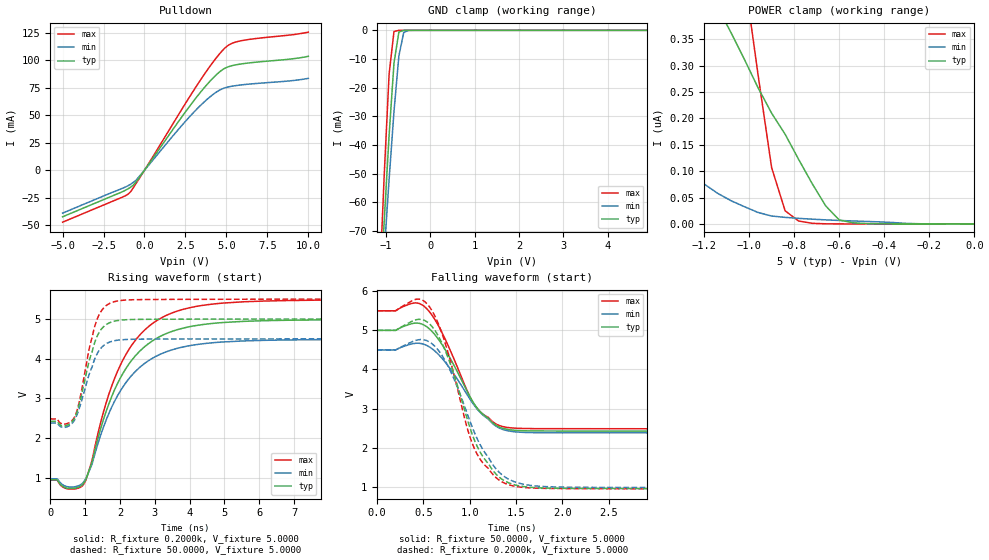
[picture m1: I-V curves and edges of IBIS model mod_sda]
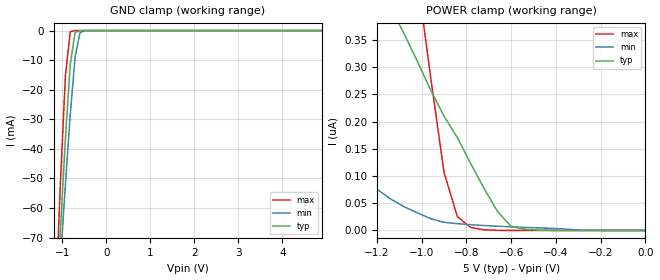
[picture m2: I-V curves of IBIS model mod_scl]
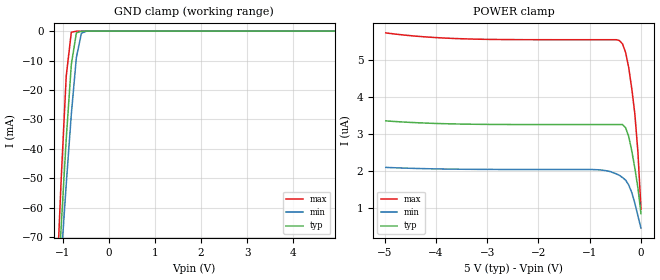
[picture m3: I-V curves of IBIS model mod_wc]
| IBIS (I/O, Buffer, Information, Specification) Model, officially
| electronic behavioral standard for Buffer structures of digital pins.
[IBIS ver]  4.0
[File name] m24512e_5d0_dfn8.ibs
[File Rev]  1.0
[Date]   26 Jan 2023
[Source]   CAD & Design Services (Catania) - STMicroelectronics
[Notes]
   (Note1)  This IBIS model includes the DFN8 package parasitic data
   (Note2)  This IBIS model has some Notes about the non-monotonicity
   of the I-V curves, but they are not indicative of problems
   inside the model;
[Disclaimer]
   Customers are solely responsible for all aspects of their
   own product designs or applications using this IBIS Model.
   STMicroelectronics assumes no liability for Custmer Designs
   and applications associated to this IBIS Model.
   In the use of this IBIS Model Customer shall not modify,
   disassemble, alter this Model in whole or in part.
   If Customers do not accept these terms, the IBIS Model
   may not be used. For any problems or modifications please
   contact STMicroelectronics (www.st.com).
[Copyright] (c) 2023 STMicroelectronics
|   Component M24512E
[Component] M24512E
[Manufacturer] STMicroelectronics
[Package]
| variable  typ   min   max
R_pkg   0.0   0.0   0.0
L_pkg   0.0H   0.0H   0.0H
C_pkg   0.0F   0.0F   0.0F
[Pin]   signal_name   model_name   R_pin   L_pin   C_pin
1   NC   NC   0.0   0.0   0.0
2   NC   NC   0.0   0.0   0.0
3   NC   NC   0.0   0.0   0.0
4   VSS   GND   0.0   0.0   0.0
5   SDA   mod_sda   0.0   0.0   0.0
6   SCL   mod_scl   0.0   0.0   0.0
7   WC   mod_wc   0.0   0.0   0.0
8   VCC   POWER   0.0   0.0   0.0
[Package Model]  182694_DFN8   | also called 182694_MLP_2x3
[Define Package Model]  182694_DFN8
[Manufacturer]  STMicroelectronics
[OEM]  STMicroelectronics
[Description]  8 pin DFN8 2x3
[Number Of Pins]  8
[Pin Numbers]
|Pin Num   Terminal Name
1   | net1
2   | net2
3   | net3
4   | net4_GND
5   | net5
6   | net6
7   | net7
8   | net8_VDD
[Model Data]
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[End Model Data]
[End Package Model]
| Models and submodels in the file (3): mod_sda (I/O_open_drain), mod_scl (Input), mod_wc (Input)
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|   Model mod_sda
[Model]   mod_sda
Model_type I/O_open_drain
Polarity   Inverting
Vinl   =   1.500V
Vinh   =   3.500V
Vmeas  =   2.500V
Cref   =   30pF
Rref   =   500
Vref   =   5.000V
C_comp   4.636pF   4.427pF   4.856pF
[Temperature Range]  25.0000   85.0000   -40.0000
[Voltage Range]   5.0000V   4.5000V   5.5000V
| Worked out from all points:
|   slope of the pulldown table from 0 to 0.75 V, typ, clamps not added: 46.8 ohm
|   GND clamp passes 1 mA (typ) near -0.71 V on its own axis
|   rising waveform, R_fixture 0.2000k, V_fixture 5.0000: 20-80 % time 1.26ns typ, 1.27ns min, 1.26ns max; typ from 0.947 V to 4.99 V
|   rising waveform, R_fixture 50.0000, V_fixture 5.0000: 20-80 % time 451ps typ, 465ps min, 432ps max; typ from 2.42 V to 5 V
|   falling waveform, R_fixture 50.0000, V_fixture 5.0000: 20-80 % time 367ps typ, 389ps min, 344ps max; typ from 5 V to 2.42 V
|   falling waveform, R_fixture 0.2000k, V_fixture 5.0000: 20-80 % time 363ps typ, 396ps min, 330ps max; typ from 5 V to 0.948 V
[Pulldown]
|Voltage   I(typ)   I(min)   I(max)
-5V       -42.42mA   -39.09mA   -47.33mA
-1.32V    -19.42mA   -16.29mA   -24.33mA
-1V       -16.92mA   -14.09mA   -21.81mA
-840mV    -15.38mA   -12.75mA   -19.46mA
-520mV    -10.86mA   -9.207mA   -12.21mA
2.04V     43.61mA    36.64mA    49.69mA
3.32V     69.2mA     57.54mA    79.96mA
4.44V     87.7mA     71.69mA    103.4mA
5.08V     94.04mA    75.73mA    113.4mA
5.4V      95.43mA    76.67mA    115.9mA
6.04V     97.07mA    77.91mA    118.3mA
10V       103.8mA    83.67mA    125.8mA
[GND_clamp]
|Voltage   I(typ)   I(min)   I(max)
-5V       -1.289A    -1.085A    -1.638A
-1.15V    -97.85mA   -103.6mA   -90.41mA
-1.04V    -66.37mA   -77.37mA   -50.31mA
-930mV    -36.57mA   -51.98mA   -15.22mA
-820mV    -11.39mA   -28.29mA   -400.6uA
-710mV    -605.6uA   -8.948mA   -4.139uA
-600mV    -10.22uA   -712.9uA   -32.48nA
-490mV    -151.4nA   -22.67uA   -140.4pA
4.9V      24.41pA    1.481nA    23.56pA
[POWER_clamp]
|Voltage   I(typ)   I(min)   I(max)
-4.98V    22.67uA    13.45uA    39.59uA
-1.92V    1.464uA    381.8nA    3.689uA
-1.74V    1.162uA    262.3nA    2.731uA
-1.14V    410.8nA    58.2nA     857.7nA
-1.08V    362.5nA    44.02nA    654.5nA
-1.02V    311.3nA    32.61nA    467.1nA
-960mV    258nA      21.75nA    282.3nA
-900mV    210nA      15.06nA    106.9nA
-840mV    170nA      12.47nA    24.93nA
-660mV    34.29nA    7.772nA    287.3pA
-600mV    7.55nA     6.641nA    82.93pA
0V        24.99pA    35.71pA    26.88pA
[Ramp]
| variable   typ   min   max
dV/dt_r   1.5460/0.4619n   1.2728/0.4770n   1.8105/0.4442n
dV/dt_f   1.5463/0.3863n   1.2731/0.4019n   1.8109/0.3591n
R_load = 50.0000
[Rising Waveform]
R_fixture= 0.2000k
V_fixture= 5.0000
V_fixture_min= 4.5000
V_fixture_max= 5.5000
|time   V(typ)   V(min)   V(max)
0s        947mV      975.4mV    941.7mV
530ps     733.1mV    770mV      716.8mV
980ps     891mV      919.3mV    862mV
1.2ns     1.396V     1.346V     1.443V
1.6ns     2.663V     2.446V     2.877V
2ns       3.494V     3.171V     3.815V
2.56ns    4.181V     3.774V     4.586V
3.22ns    4.588V     4.134V     5.04V
4.95ns    4.908V     4.419V     5.397V
10ns      4.988V     4.489V     5.488V
[Rising Waveform]
R_fixture= 50.0000
V_fixture= 5.0000
V_fixture_min= 4.5000
V_fixture_max= 5.5000
|time   V(typ)   V(min)   V(max)
0s        2.422V     2.378V     2.482V
200ps     2.422V     2.378V     2.482V
390ps     2.303V     2.267V     2.35V
700ps     2.51V      2.459V     2.534V
840ps     2.879V     2.766V     2.943V
1.1ns     3.885V     3.562V     4.177V
1.3ns     4.467V     4.042V     4.88V
1.5ns     4.777V     4.306V     5.243V
1.78ns    4.929V     4.438V     5.418V
10ns      4.999V     4.499V     5.499V
[Falling Waveform]
R_fixture= 50.0000
V_fixture= 5.0000
V_fixture_min= 4.5000
V_fixture_max= 5.5000
|time   V(typ)   V(min)   V(max)
0s        5V         4.5V       5.5V
200ps     5V         4.5V       5.5V
410ps     5.185V     4.668V     5.701V
520ps     5.117V     4.631V     5.589V
720ps     4.565V     4.231V     4.849V
980ps     3.407V     3.327V     3.414V
1.06ns    3.079V     3.049V     3.065V
1.26ns    2.614V     2.592V     2.644V
1.42ns    2.465V     2.431V     2.515V
10ns      2.423V     2.378V     2.482V
[Falling Waveform]
R_fixture= 0.2000k
V_fixture= 5.0000
V_fixture_min= 4.5000
V_fixture_max= 5.5000
|time   V(typ)   V(min)   V(max)
0s        5V         4.5V       5.5V
200ps     5V         4.5V       5.5V
430ps     5.276V     4.753V     5.798V
560ps     5.177V     4.71V      5.618V
760ps     4.339V     4.114V     4.478V
960ps     2.837V     2.956V     2.615V
1.06ns    2.144V     2.337V     1.93V
1.28ns    1.337V     1.473V     1.246V
1.48ns    1.057V     1.134V     1.021V
10ns      948.2mV    977mV      942.7mV
|   Model mod_scl
[Model]   mod_scl
Model_type Input
Vinl   =   1.500V
Vinh   =   3.500V
C_comp   3.207pF   3.063pF   3.358pF
[Temperature Range]  25.0000   85.0000   -40.0000
[Voltage Range]   5.0000V   4.5000V   5.5000V
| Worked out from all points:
|   GND clamp passes 1 mA (typ) near -0.71 V on its own axis
[GND_clamp]
|Voltage   I(typ)   I(min)   I(max)
-5V       -1.289A    -1.085A    -1.638A
-1.15V    -97.85mA   -103.6mA   -90.41mA
-1.04V    -66.37mA   -77.37mA   -50.31mA
-930mV    -36.57mA   -51.98mA   -15.22mA
-820mV    -11.39mA   -28.29mA   -400.6uA
-710mV    -605.6uA   -8.948mA   -4.139uA
-600mV    -10.22uA   -712.9uA   -32.48nA
-490mV    -151.4nA   -22.67uA   -140.4pA
4.9V      24.41pA    1.481nA    23.56pA
[POWER_clamp]
|Voltage   I(typ)   I(min)   I(max)
-4.98V    22.67uA    13.45uA    39.59uA
-1.92V    1.464uA    381.8nA    3.689uA
-1.74V    1.162uA    262.3nA    2.731uA
-1.14V    410.8nA    58.2nA     857.7nA
-1.08V    362.5nA    44.02nA    654.5nA
-1.02V    311.3nA    32.61nA    467.1nA
-960mV    258nA      21.75nA    282.3nA
-900mV    210nA      15.06nA    106.9nA
-840mV    170nA      12.47nA    24.93nA
-660mV    34.29nA    7.772nA    287.3pA
-600mV    7.55nA     6.641nA    82.93pA
0V        24.99pA    35.71pA    26.88pA
|   Model mod_wc
[Model]   mod_wc
Model_type Input
Vinl   =   1.500V
Vinh   =   3.500V
C_comp   3.207pF   3.063pF   3.358pF
[Temperature Range]  25.0000   85.0000   -40.0000
[Voltage Range]   5.0000V   4.5000V   5.5000V
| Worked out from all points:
|   GND clamp passes 1 mA (typ) near -0.71 V on its own axis
[GND_clamp]
|Voltage   I(typ)   I(min)   I(max)
-5V       -1.289A    -1.085A    -1.638A
-1.15V    -97.85mA   -103.6mA   -90.41mA
-1.04V    -66.37mA   -77.37mA   -50.32mA
-930mV    -36.57mA   -51.98mA   -15.23mA
-820mV    -11.4mA    -28.29mA   -412.6uA
-710mV    -614.3uA   -8.95mA    -18.98uA
-600mV    -21.18uA   -719.3uA   -12.14uA
-490mV    -9.233uA   -30.85uA   -9.572uA
4.9V      4.249uA    2.039uA    6.534uA
[POWER_clamp]
|Voltage   I(typ)   I(min)   I(max)
-4.98V    3.349uA    2.096uA    5.718uA
-3.54V    3.264uA    2.047uA    5.562uA
-960mV    3.249uA    2.039uA    5.534uA
-600mV    3.249uA    1.983uA    5.534uA
-420mV    3.249uA    1.882uA    5.511uA
-360mV    3.249uA    1.821uA    5.42uA
-300mV    3.163uA    1.753uA    5.192uA
-240mV    2.93uA     1.622uA    4.788uA
-180mV    2.542uA    1.42uA     4.222uA
-120mV    2.077uA    1.132uA    3.538uA
-60mV     1.543uA    789nA      2.511uA
0V        849.4nA    459.1nA    970nA
